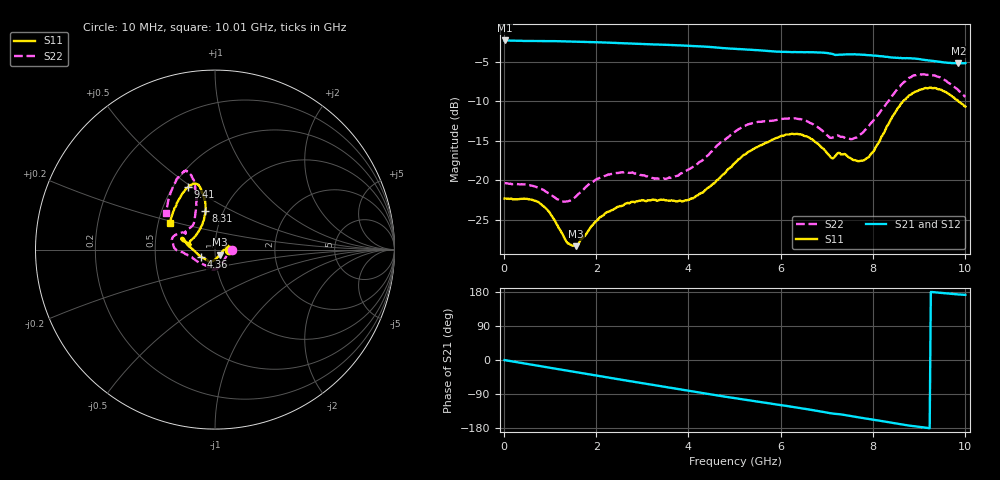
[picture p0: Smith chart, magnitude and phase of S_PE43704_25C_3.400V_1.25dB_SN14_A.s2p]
! Device ID: PE43704
! Dir: z:\PE43704\PE43704_Char_1_20130516\PE43704\AMB\3p400V\1p25dB
! Serial: 14
! Insertion: A
! Impedance: 50 ohm
! Temp: Amb
! VDD: 3.400V
! Attenuation Step: 1.25dB
! IDD: 1.140926e-01mA
#  Hz  S  RI  R  50
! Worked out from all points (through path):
!   401 points, 10 MHz to 10.01 GHz, reference 50 ohm
!   highest |S21| = -2.28 dB at 10 MHz (marker M1); lowest = -5.2 dB at 9.86 GHz (marker M2)
!   group delay of S21, straight-line fit = 53.5 ps
!   lowest |S11| = -28.3 dB at 1.56 GHz (marker M3), VSWR 1.08, Z = 52.5 - j3 ohm
!   |S11| at or under -10 dB: start of sweep to 8.656 GHz; 9.859 GHz to end of sweep
!   |S22| runs from -22.7 to -6.6 dB; largest |S21 - S12| = 0.0054
!   S11 on the Smith chart (normalised r, x): 10 MHz: 1.17, +0.00; 4.36 GHz: 0.86, -0.07; 8.31 GHz: 0.82, +0.37; 9.41 GHz: 0.59, +0.48; 10.01 GHz: 0.58, +0.19
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1e7  0.0766 0.000308  0.769 -0.00326  0.769 -0.00318  0.0961 0.000102
7.6e8  0.069 0.0211  0.7342 -0.2055  0.7341 -0.2054  0.0889 0.00698
1.26e9  0.0455 -0.00483  0.6833 -0.3323  0.6834 -0.3321  0.0667 -0.0307
1.56e9  0.0255 -0.0285  0.641 -0.402  0.6408 -0.402  0.0489 -0.0621
1.685e9  0.0178 -0.0386  0.6207 -0.4299  0.6208 -0.4298  0.0402 -0.0752
2.035e9  -0.000932 -0.0565  0.558 -0.4995  0.5583 -0.4995  0.0196 -0.1006
2.46e9  -0.0179 -0.0655  0.472 -0.5708  0.4726 -0.5706  -0.00518 -0.1111
3.36e9  -0.0288 -0.0691  0.2682 -0.6725  0.2689 -0.6721  -0.0384 -0.0948
3.91e9  -0.0476 -0.0569  0.1332 -0.7007  0.1338 -0.7007  -0.0862 -0.0732
4.36e9  -0.0762 -0.0412  0.0206 -0.702  0.0212 -0.7029  -0.1337 -0.0407
5.01e9  -0.1288 0.00476  -0.1281 -0.6682  -0.1279 -0.6684  -0.2031 -0.00887
6.035e9  -0.1806 0.0644  -0.3208 -0.567  -0.3184 -0.5681  -0.2397 0.0503
6.685e9  -0.1759 0.0462  -0.4338 -0.4809  -0.4346 -0.48  -0.2109 0.0868
7.085e9  -0.1366 0.0305  -0.4892 -0.4049  -0.4914 -0.4058  -0.163 0.0895
7.76e9  -0.1008 0.0879  -0.5551 -0.2863  -0.5549 -0.2875  -0.1153 0.161
7.985e9  -0.0783 0.1274  -0.5701 -0.2402  -0.5702 -0.243  -0.1089 0.2075
8.31e9  -0.0533 0.2142  -0.5805 -0.1736  -0.5782 -0.1762  -0.1059 0.2916
8.36e9  -0.0522 0.2268  -0.5803 -0.1615  -0.5793 -0.1649  -0.1046 0.3066
8.835e9  -0.0805 0.3404  -0.5888 -0.0637  -0.5849 -0.0647  -0.1443 0.4268
9.41e9  -0.1489 0.3476  -0.5646 0.023  -0.5642 0.0242  -0.202 0.4057
9.86e9  -0.2292 0.2175  -0.5471 0.0675  -0.5456 0.0689  -0.262 0.2628
1.001e10  -0.252 0.1496  -0.5473 0.0783  -0.5505 0.0786  -0.2717 0.2014
